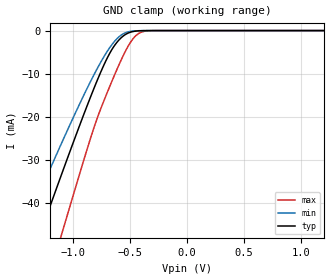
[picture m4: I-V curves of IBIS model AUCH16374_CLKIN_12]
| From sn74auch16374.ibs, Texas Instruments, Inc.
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[Model]   AUCH16374_CLKIN_12
Model_type  Input
Vinl=0.385
Vinh=0.845
| variable   typ   min   max
C_comp   2.51pF   2.11pF   2.87pF
[Temperature Range]   40   100   -40
| Ambient temperature   25   85   -40
[Voltage range]   1.2   1.1   1.3
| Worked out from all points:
|   GND clamp passes 1 mA (typ) near -0.55 V on its own axis
[GND Clamp]
| AUCH16374_CLKIN_12
|   Voltage   I(typ)   I(min)   I(max)
-3.6V     -222.3mA   -186.1mA   -267.5mA
-1.445V   -58.91mA   -46.99mA   -78.09mA
-1.275V   -46.22mA   -36.57mA   -62.93mA
-1.11V    -34.06mA   -26.69mA   -48.19mA
-1.075V   -31.52mA   -24.64mA   -45.06mA
-835mV    -14.65mA   -11.22mA   -24.05mA
-695mV    -6.114mA   -4.621mA   -14.06mA
-575mV    -1.603mA   -998.8uA   -6.664mA
-500mV    -407.1uA   -201.6uA   -2.896mA
-440mV    -95.43uA   -45.03uA   -977.4uA
-320mV    -2.85uA    -1.742uA   -25.53uA
1.2V      133.3pA    223pA      123.7pA
